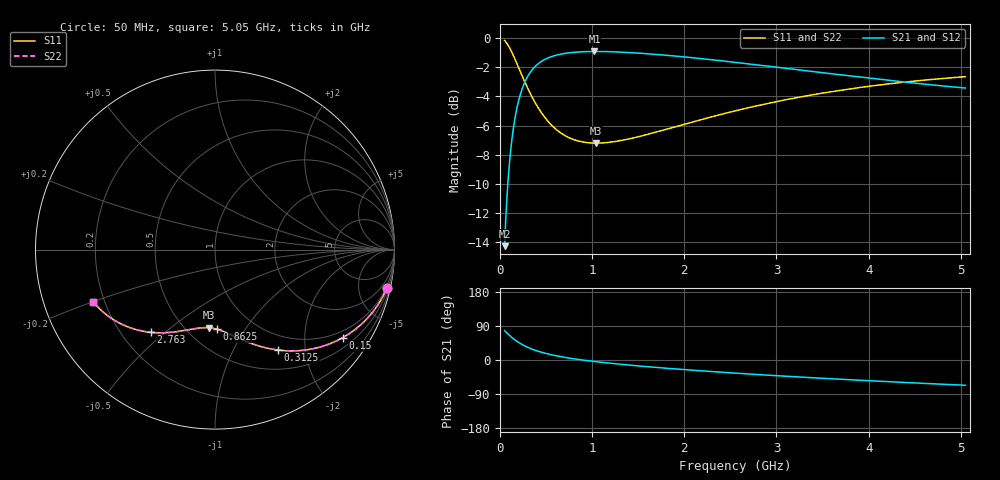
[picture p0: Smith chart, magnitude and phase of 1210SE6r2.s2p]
! AVX Thin Film Operation		Date: August 2001
! Description: Accu-P® Series, Thin Film, SMD, RF Capacitor
! Part Number: 12101J6R2BBT
! 50 MHz  -  5.05 GHz
! Serial Measurements
# mhz S db R 50
!	S11		S21		S12		S22
!	dB	Phase	dB	Phase	dB	Phase	dB	Phase
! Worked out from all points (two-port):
!   401 points, 50 MHz to 5.05 GHz, reference 50 ohm
!   highest |S21| = -0.92 dB at 1.025 GHz (marker M1); lowest = -14.3 dB at 50 MHz (marker M2)
!   |S21| within 3 dB of the highest: 217.9 MHz to end of sweep
!   lowest |S11| = -7.2 dB at 1.038 GHz (marker M3), VSWR 2.55, Z = 32.2 - j34.7 ohm
!   |S11| at or under -10 dB: nowhere
!   |S22| runs from -7.2 to -0.2 dB; largest |S21 - S12| = 0
!   S11 on the Smith chart (normalised r, x): 50 MHz: 0.78, -8.95; 150 MHz: 0.78, -3.03; 312.5 MHz: 0.77, -1.53; 862.5 MHz: 0.68, -0.75; 2.763 GHz: 0.32, -0.45; 5.05 GHz: 0.16, -0.20
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50  -0.17 -12.7  -14.25 77.3  -14.25 77.3  -0.17 -12.7
75  -0.36 -18.7  -10.96 71.3  -10.96 71.3  -0.36 -18.7
100  -0.62 -24.4  -8.75 65.6  -8.75 65.6  -0.62 -24.4
150  -1.27 -34.6  -5.97 55.4  -5.97 55.4  -1.27 -34.6
187.5  -1.81 -41.3  -4.68 48.7  -4.68 48.7  -1.81 -41.3
225  -2.37 -47.0  -3.77 42.9  -3.77 42.9  -2.37 -47.0
312.5  -3.60 -57.8  -2.50 32.1  -2.50 32.1  -3.60 -57.8
412.5  -4.76 -66.8  -1.77 23.1  -1.77 23.1  -4.76 -66.8
525  -5.73 -74.3  -1.35 15.6  -1.35 15.6  -5.73 -74.3
675  -6.57 -81.8  -1.08 8.2  -1.08 8.2  -6.57 -81.8
862.5  -7.07 -88.9  -0.95 1.1  -0.95 1.1  -7.07 -88.9
887.5  -7.11 -89.7  -0.94 0.2  -0.94 0.2  -7.11 -89.7
1025  -7.20 -93.9  -0.92 -4.0  -0.92 -4.0  -7.20 -93.9
1037.5  -7.20 -94.3  -0.92 -4.3  -0.92 -4.3  -7.20 -94.3
1350  -6.97 -102.2  -0.98 -12.2  -0.98 -12.2  -6.97 -102.2
1725  -6.39 -110.2  -1.14 -20.2  -1.14 -20.2  -6.39 -110.2
2125  -5.69 -117.6  -1.37 -27.6  -1.37 -27.6  -5.69 -117.6
2550  -4.99 -124.6  -1.66 -34.6  -1.66 -34.6  -4.99 -124.6
2762.5  -4.68 -127.9  -1.82 -37.9  -1.82 -37.9  -4.67 -127.9
3387.5  -3.89 -136.8  -2.29 -46.8  -2.29 -46.8  -3.89 -136.8
4225  -3.13 -147.3  -2.90 -57.3  -2.90 -57.3  -3.13 -147.3
5050  -2.65 -156.7  -3.42 -66.7  -3.42 -66.7  -2.65 -156.7
